FUNCTION_BLOCK PUBLIC GetMeasure
VAR_INPUT
	nominalMeasure   : UDINT;
	variance         : UDINT;
	steps            : UINT;
END_VAR
VAR_OUTPUT
	measure           : UDINT;
END_VAR
VAR
	FB_SystemTime    : GETSYSTEMTIME;
	currTimeLo       : UDINT;
	currTimeHi       : UDINT;
	
	FB_Randomizer    : DRAND;
	rand             : LREAL;
	seed             : INT;	

	varianceEffective: UDINT;
	varianceAbsolute : UDINT;
	deviation        : UDINT;	
END_VAR

FB_SystemTime( timeLoDW => currTimeLo, timeHiDW => currTimeHi );
seed := UDINT_TO_INT(currTimeLo);
FB_Randomizer(Seed := seed, Num => rand);
varianceEffective := variance / steps;

varianceAbsolute := LREAL_TO_UINT(rand * UDINT_TO_LREAL(varianceEffective)) * steps;

IF varianceAbsolute >= (variance / 2) THEN
	deviation := varianceAbsolute - (variance / 2);	
	measure := nominalMeasure + deviation;
ELSE
	deviation := (variance / 2) - varianceAbsolute;
	measure := nominalMeasure - deviation;
END_IF

END_FUNCTION_BLOCK
